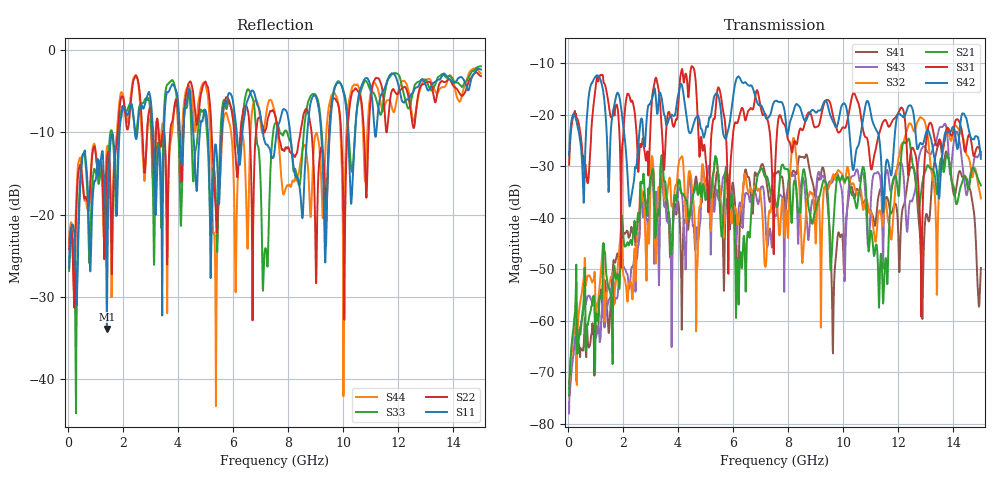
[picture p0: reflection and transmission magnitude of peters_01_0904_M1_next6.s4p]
# MHZ S RI R 50.00
! FREQ  S11  S12  S13  S14
!  S21  S22  S23  S24
!  S31  S32  S33  S34
!  S41  S42  S43  S44
!  REAL  IMAG  REAL  IMAG  REAL  IMAG  REAL  IMAG
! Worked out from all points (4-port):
!   1496 points, 50 MHz to 15 GHz, reference 50 ohm
!   strongest paths, dB at 50 MHz, 3.79 GHz, 7.53 GHz, 11.27 GHz, 15 GHz:
!     S42: -28.0, -20.0, -17.3, -23.6, -28.6
!     S31: -29.7, -21.3, -30.5, -24.4, -27.9
!     S21: -74.6, -45.4, -36.8, -50.7, -33.7
!     S32: -72.2, -37.5, -36.5, -39.5, -36.2
!     S43: -78.0, -54.1, -39.5, -31.2, -27.2
!     S41: -73.2, -46.1, -31.4, -36.2, -49.8
!   lowest |S11| = -33.9 dB at 1.42 GHz (marker M1), VSWR 1.04, Z = 48.7 - j1.48 ohm
!   |S11| at or under -10 dB: start of sweep to 1.879 GHz; 5.089 GHz to 5.587 GHz (498.5 MHz wide, 9.34 % of centre); 8.074 GHz to 8.698 GHz (624.3 MHz wide, 7.44 % of centre)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
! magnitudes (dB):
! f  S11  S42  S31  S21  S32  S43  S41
! 50 MHz  -26.5  -28.0  -29.7  -74.6  -72.2  -78.0  -73.2
! 1.42 GHz  -33.9  -24.2  -15.9  -51.8  -54.5  -57.7  -56.8
! 4.11 GHz  -13.0  -14.0  -11.9  -34.9  -28.3  -34.9  -49.1
! 8.47 GHz  -18.4  -19.1  -22.7  -36.9  -42.4  -33.4  -28.2
! 12.87 GHz  -3.6  -25.8  -42.3  -33.4  -20.7  -26.5  -59.6
! 13.49 GHz  -3.6  -36.1  -24.8  -30.8  -33.3  -22.6  -25.4
! 15 GHz  -2.4  -28.6  -27.9  -33.7  -36.2  -27.2  -49.8
